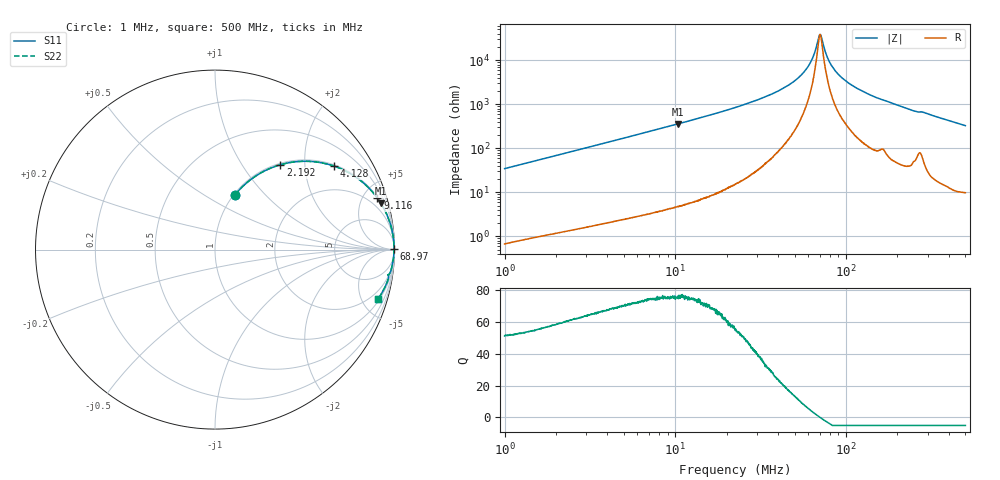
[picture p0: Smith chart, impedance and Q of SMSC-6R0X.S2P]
!s-Parameter Generated by FASTRON Sdn. Bhd.
!FASTRON P/N : SMSC-6R0X
!Keysight Technologies,E4991B,MY54100416,A.01.15
!Date: Mon Mar 16 10:15:10 2026
!Version  : Rev00 Mon Mar 16 10:15:10 2026
!Data & Calibration Information:
!PortZ  Port1:50+j0  Port2:50+j0
!When reading, reference impedance value at option line is always used.
!Remarks : This data is being provided solely for informational purposes.
!Freq	S11	S21	S12	S22
# Hz S dB R 50
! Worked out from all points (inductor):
!   1601 points, 1 MHz to 500 MHz, reference 50 ohm
!   read as one part in series: L = 5.49 uH near 1.032 MHz
!   highest Q = 76 at 10.32 MHz (marker M1), where L = 5.51 uH
!   self-resonance near 70.32 MHz
!   S11 on the Smith chart (normalised r, x): 1 MHz: 1.01, +0.69; 2.192 MHz: 1.03, +1.50; 4.128 MHz: 1.04, +2.82; 9.116 MHz: 1.08, +6.29; 68.97 MHz: open; 500 MHz: 1.20, -6.55
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1000000  -9.76 69.9  -0.54 -19.0  -0.54 -19.0  -9.76 69.9
2191518  -4.49 52.4  -2.02 -36.6  -2.02 -36.6  -4.49 52.4
2820919  -3.23 45.5  -2.93 -43.6  -2.93 -43.6  -3.23 45.5
4127647  -1.83 35.0  -4.82 -54.1  -4.82 -54.1  -1.83 35.0
7957584  -0.58 20.0  -9.32 -69.2  -9.32 -69.2  -0.58 20.0
9116355  -0.45 17.6  -10.40 -71.7  -10.40 -71.7  -0.45 17.6
1.032287e7  -0.36 15.6  -11.42 -73.7  -11.42 -73.7  -0.36 15.6
2.236068e7  -0.08 6.8  -18.58 -82.2  -18.58 -82.2  -0.08 6.8
3.401461e7  -0.04 3.8  -23.58 -84.4  -23.58 -84.4  -0.04 3.8
4.551764e7  -0.03 2.2  -28.48 -84.5  -28.48 -84.5  -0.03 2.2
5.548932e7  -0.02 1.2  -33.87 -82.3  -33.87 -82.3  -0.02 1.2
6.307767e7  -0.02 0.5  -40.34 -74.7  -40.34 -74.7  -0.02 0.5
6.897208e7  -0.02 0.1  -50.11 -35.8  -50.11 -35.8  -0.02 0.1
7.032465e7  -0.02 0.0  -51.74 -4.5  -51.74 -4.5  -0.02 0.0
7.142578e7  -0.02 -0.1  -51.04 23.0  -51.04 23.0  -0.02 -0.1
7.659818e7  -0.02 -0.4  -42.62 68.2  -42.62 68.2  -0.02 -0.4
8.02529e7  -0.02 -0.6  -39.05 75.1  -39.05 75.1  -0.02 -0.6
8.639945e7  -0.03 -1.0  -35.25 79.8  -35.25 79.8  -0.03 -1.0
9.484087e7  -0.03 -1.4  -31.97 81.9  -31.97 81.9  -0.03 -1.4
1.239906e8  -0.04 -2.8  -26.08 83.1  -26.08 83.1  -0.04 -2.8
1.77937e8  -0.08 -5.0  -21.15 81.8  -21.15 81.8  -0.08 -5.0
5e8  -0.46 -16.8  -10.76 71.5  -10.76 71.5  -0.46 -16.8
